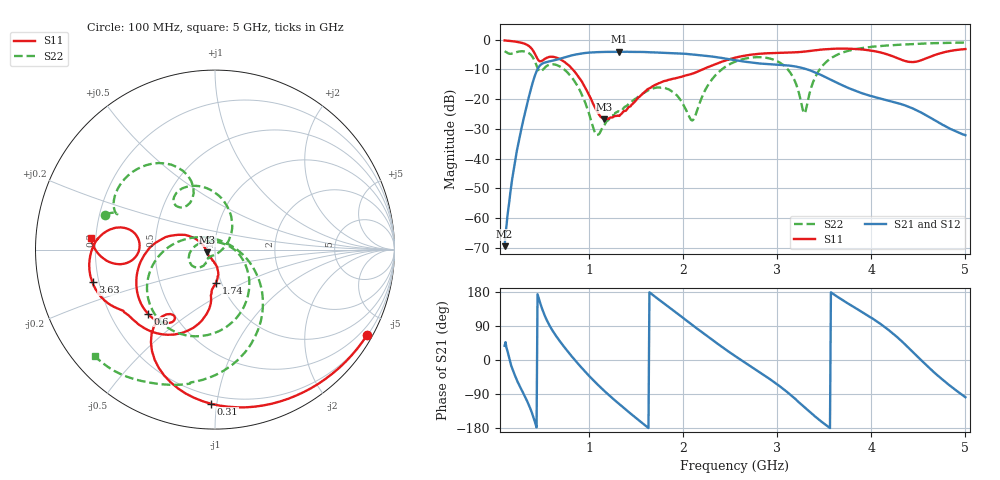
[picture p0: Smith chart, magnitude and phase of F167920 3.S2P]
!  2-Port S-parameters saved by WinCal
! VAR MeasName=S-Parameters (CALIBRATED_DATA) read from VNA (N5242A)
! VAR MeasDate=2016-11-22 9:53:33
! VAR NAME=F167920 3
! VAR FILENAME=F167920 3.S2P
! VAR DATE=2016-11-22 9:53:33
! VAR PHYS_PORTS=1,2
# Hz S DB R 50
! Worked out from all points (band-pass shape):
!   491 points, 100 MHz to 5 GHz, reference 50 ohm
!   highest |S21| = -4.03 dB at 1.32 GHz (marker M1); lowest = -69.5 dB at 100 MHz (marker M2)
!   |S21| within 3 dB of the highest: 615.4 MHz to 2.578 GHz (1.962 GHz wide, 123 % of centre)
!   lowest |S11| = -26.8 dB at 1.16 GHz (marker M3), VSWR 1.10, Z = 45.8 - j1.33 ohm
!   |S11| at or under -10 dB: 823.2 MHz to 2.207 GHz (1.384 GHz wide, 91.3 % of centre)
!   |S22| runs from -32.1 to -1.0 dB; largest |S21 - S12| = 0.0017
!   S11 on the Smith chart (normalised r, x): 100 MHz: 0.22, -3.82; 310 MHz: 0.15, -0.96; 600 MHz: 0.36, -0.35; 1.74 GHz: 0.94, -0.36; 3.63 GHz: 0.17, -0.13; 5 GHz: 0.18, +0.05
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1e8  -0.25 -29.3  -69.52 37.4  -69.66 56.5  -3.86 162.5
2e8  -0.58 -58.0  -42.99 -35.1  -42.94 -35.2  -4.47 159.0
3.1e8  -1.31 -91.5  -25.55 -93.2  -25.56 -93.1  -3.93 139.3
3.9e8  -3.10 -118.7  -15.41 -139.0  -15.40 -139.0  -5.48 117.2
4.7e8  -7.20 -124.7  -8.89 157.0  -8.89 157.0  -10.61 118.1
6e8  -5.74 -136.4  -7.15 81.5  -7.14 81.5  -8.26 120.3
9.2e8  -14.01 155.4  -4.60 -20.8  -4.60 -20.8  -18.48 42.5
1.07e9  -23.41 162.1  -4.21 -60.2  -4.20 -60.2  -31.80 -42.3
1.16e9  -26.79 -161.5  -4.11 -81.6  -4.11 -81.6  -28.74 -113.5
1.32e9  -25.67 -114.6  -4.03 -116.5  -4.03 -116.5  -24.17 -130.1
1.74e9  -14.64 -88.5  -4.35 159.5  -4.35 159.5  -16.08 -150.7
2.1e9  -11.39 -94.7  -4.96 91.6  -4.95 91.6  -27.14 71.8
2.29e9  -8.87 -97.3  -5.59 56.6  -5.58 56.6  -14.00 -29.0
2.55e9  -6.06 -111.4  -6.88 10.6  -6.88 10.6  -7.41 -79.3
3.01e9  -4.44 -139.0  -8.45 -66.3  -8.43 -66.4  -7.41 -152.6
3.17e9  -4.28 -144.6  -8.88 -98.1  -8.86 -98.2  -12.81 171.6
3.28e9  -4.03 -148.2  -9.64 -122.7  -9.61 -122.8  -24.55 88.8
3.37e9  -3.69 -151.5  -10.58 -142.3  -10.55 -142.5  -15.17 -14.0
3.63e9  -3.02 -165.0  -14.43 168.3  -14.41 168.1  -5.17 -67.6
4.19e9  -5.15 167.1  -20.59 77.8  -20.63 77.7  -1.90 -110.8
4.64e9  -5.56 -171.2  -26.48 -26.2  -26.50 -26.6  -1.19 -127.9
5e9  -3.15 174.7  -32.16 -98.3  -32.18 -98.7  -0.96 -138.4
